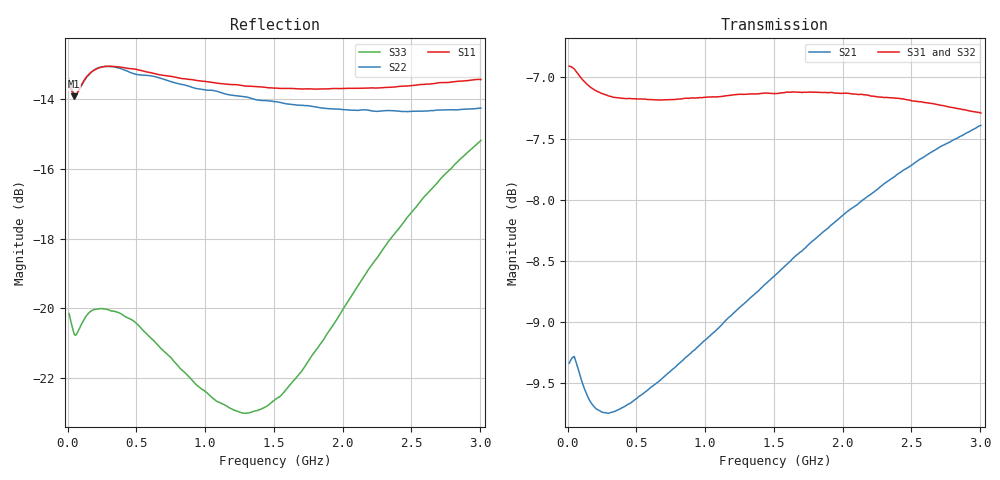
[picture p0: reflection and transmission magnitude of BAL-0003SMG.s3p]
! MARKI MICROWAVE INC.
! Email:  info@markimicrowave.com  Phone:  408-778-4200
! Model Number:  BAL-0003SM  Date:  12/12
! Filename:		BAL-0003SM.S3P  Version: 1.0
! Description:  3-port S-parameter data for Balun BAL-0003SM
! Frequency Range: 	10 MHz to 3 GHz
! Port Configuration:	PORT 1: OUTPUT (0 DEGREE), PORT 2: OUTPUT (180 DEGREE), PORT 3:COMMON
! S3P File: Measurements: Mag<S11> Ang<S11> Mag<S12> Ang<S12> Mag<S13> Ang<S13>! row 1
!  Mag<S21> Ang<S21> Mag<S22> Ang<S22> Mag<S23> Ang<S23>! row 2
!  Mag<S31> Ang<S31> Mag<S32> Ang<S32> Mag<S33> Ang<S33>! row 3
# Hz S  dB  R 50
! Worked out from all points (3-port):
!   401 points, 10 MHz to 3.005 GHz, reference 50 ohm
!   strongest paths, dB at 10 MHz, 758.8 MHz, 1.508 GHz, 2.256 GHz, 3.005 GHz:
!     S31: -6.9, -7.2, -7.1, -7.2, -7.3
!     S32: -7.0, -7.2, -7.2, -7.2, -7.2
!     S21: -9.3, -9.4, -8.6, -7.9, -7.4
!   lowest |S11| = -13.9 dB at 47.44 MHz (marker M1), VSWR 1.50, Z = 33.3 + j1.51 ohm
!   |S11| at or under -10 dB: start of sweep to end of sweep
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1e7  -13.56 166.4  -9.33 5.0  -6.90 -0.7
     -9.34 4.4  -13.43 165.5  -6.95 179.7
     -6.91 0.2  -6.98 -179.0  -20.15 165.0
4.74375e7  -13.92 173.8  -9.30 -2.5  -6.92 -4.2
           -9.28 -2.5  -13.90 173.2  -6.93 175.9
           -6.93 -4.4  -6.95 175.7  -20.75 173.4
4.5925e8  -13.12 143.6  -9.67 -31.2  -7.16 -41.5
          -9.66 -31.1  -13.24 142.1  -7.20 137.6
          -7.17 -41.4  -7.21 137.7  -20.32 150.4
8.1865e8  -13.40 115.4  -9.34 -55.7  -7.17 -73.3
          -9.33 -55.6  -13.57 112.7  -7.21 105.3
          -7.18 -73.1  -7.23 105.5  -21.73 131.6
1.155588e9  -13.57 90.2  -8.99 -79.8  -7.14 -103.3
            -8.98 -79.7  -13.85 86.8  -7.20 74.9
            -7.15 -103.1  -7.22 75.0  -22.81 121.7
1.5075e9  -13.68 64.5  -8.63 -105.6  -7.12 -135.0
          -8.62 -105.6  -14.07 60.4  -7.19 43.0
          -7.13 -134.8  -7.20 43.1  -22.63 117.3
1.851925e9  -13.70 39.8  -8.27 -131.7  -7.12 -166.0
            -8.27 -131.6  -14.25 35.4  -7.17 11.7
            -7.12 -165.9  -7.18 11.8  -20.95 107.6
2.188862e9  -13.68 16.4  -7.97 -157.6  -7.15 163.5
            -7.97 -157.5  -14.32 11.6  -7.17 -18.9
            -7.15 163.7  -7.18 -18.8  -18.88 90.3
2.623138e9  -13.57 -13.7  -7.64 168.4  -7.20 124.2
            -7.63 168.6  -14.33 -18.2  -7.17 -58.3
            -7.21 124.4  -7.19 -58.2  -16.67 60.7
3.005e9  -13.43 -39.5  -7.40 138.2  -7.28 89.8
         -7.39 138.3  -14.25 -43.3  -7.20 -92.8
         -7.29 89.9  -7.22 -92.7  -15.18 30.7
